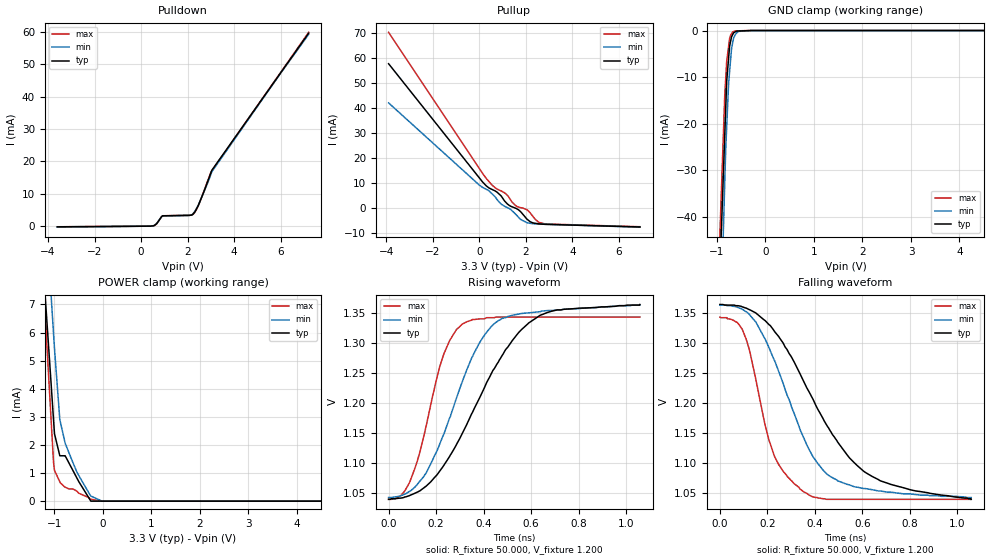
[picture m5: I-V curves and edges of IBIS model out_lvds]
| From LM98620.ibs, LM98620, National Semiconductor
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[Model] out_lvds
Model_type Output
Vref=1.20000V
Rref=50.0000ohms
Cref=0.00000F
Vmeas=1.20000V
C_comp 737.000fF 691.000fF 817.000fF
| variable typ   min   max
[Voltage Range] 3.30000V 3.00000V 3.60000V
[POWER Clamp Reference] 3.30000V 3.00000V 3.60000V
[Pullup Reference] 3.30000V 3.00000V 3.60000V
[Pulldown Reference] 0.00000V 0.00000V 0.00000V
[GND Clamp Reference] 0.00000V 0.00000V 0.00000V
[Temperature Range]   25   70   0
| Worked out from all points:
|   slope of the pulldown table from 0 to 0.495 V, typ, clamps not added: 4.65 kohm
|   slope of the pullup table from 0 to 0.495 V, typ, clamps not added: 113 ohm
|   GND clamp passes 1 mA (typ) near -0.68 V on its own axis
|   POWER clamp passes 1 mA (typ) near -0.59 V on its own axis
|   rising waveform, R_fixture 50.000, V_fixture 1.200: 20-80 % time 266ps typ, 194ps min, 115ps max; typ from 1.04 V to 1.36 V
|   falling waveform, R_fixture 50.000, V_fixture 1.200: 20-80 % time 289ps typ, 200ps min, 116ps max; typ from 1.36 V to 1.04 V
[GND Clamp]
-3.6V     -828.7mA   -1.023A    -833.8mA
-3V       -653.4mA   -808mA     -655.6mA
-840mV    -22.57mA   -32.76mA   -14mA
-820mV    -16.73mA   -25.58mA   -10.34mA
-800mV    -10.89mA   -20.83mA   -6.68mA
-760mV    -5.872mA   -11.32mA   -3.357mA
-740mV    -3.363mA   -8.853mA   -1.695mA
-700mV    -1.363mA   -3.922mA   -701.6uA
-660mV    -522.6uA   -1.717mA   -216.5uA
-560mV    -109.8uA   -188.4uA   -61.51uA
-280mV    0A         0A         0A
7.2V      0A         0A         0A
[Pulldown]
-3.6V     -228.1uA   -333.2uA   -216.3uA
400mV     -26.54uA   -21.17uA   -29.46uA
540mV     100.7uA    166uA      76.81uA
680mV     832uA      952.1uA    779.9uA
920mV     3.176mA    3.133mA    3.192mA
2.06V     3.322mA    3.282mA    3.336mA
2.22V     3.619mA    3.762mA    3.559mA
2.34V     4.764mA    4.947mA    4.614mA
2.5V      7.154mA    7.187mA    6.982mA
3V        16.5mA     16.05mA    16.71mA
3.04V     17.27mA    16.85mA    17.12mA
7.2V      59.7mA     59.34mA    59.95mA
[Pullup]
-3.9V     57.71mA    42.03mA    70.29mA
0V        12mA       9.116mA    15.74mA
260mV     9.187mA    7.62mA     12.25mA
420mV     7.937mA    6.794mA    10.47mA
760mV     6.288mA    3.336mA    7.56mA
1.12V     2.406mA    487.7uA    5.771mA
1.58V     -213.1uA   -2.707mA   748.1uA
1.78V     -1.58mA    -4.658mA   76.77uA
2.18V     -5.52mA    -6.172mA   -1.952mA
2.52V     -6.367mA   -6.468mA   -5.559mA
2.8V      -6.573mA   -6.548mA   -6.373mA
6.9V      -7.647mA   -7.716mA   -7.544mA
[POWER Clamp]
-3.9V     76.64mA    84.41mA    106.3mA
-1.3V     10.08mA    13.6mA     10.8mA
-1.16V    6.495mA    9.79mA     5.659mA
-1.02V    2.911mA    5.977mA    1.391mA
-1V       2.399mA    5.433mA    1.094mA
-890mV    1.615mA    2.904mA    689.6uA
-780mV    1.615mA    2.062mA    496.3uA
-540mV    829.4uA    1.046mA    358.3uA
-500mV    698.5uA    914.1uA    282.6uA
-250mV    0A         180.7uA    65.92uA
-20mV     0A         0A         0A
6.9V      0A         0A         0A
[Rising Waveform]
R_fixture = 50.000
V_fixture = 1.200
V_fixture_min = 1.200
V_fixture_max = 1.200
|  time   V(typ)   V(min)   V(max)
0s        1.04V      1.043V     1.04V
87ps      1.046V     1.053V     1.067V
155ps     1.061V     1.082V     1.157V
233ps     1.097V     1.149V     1.283V
309ps     1.149V     1.235V     1.332V
360ps     1.191V     1.284V     1.34V
429ps     1.247V     1.327V     1.343V
589ps     1.334V     1.351V     1.344V
710ps     1.356V     1.356V     1.344V
1.058ns   1.365V     1.364V     1.344V
[Falling Waveform]
R_fixture = 50.000
V_fixture = 1.200
V_fixture_min = 1.200
V_fixture_max = 1.200
|  time   V(typ)   V(min)   V(max)
0s        1.365V     1.364V     1.344V
94ps      1.361V     1.357V     1.324V
151ps     1.351V     1.336V     1.241V
191ps     1.338V     1.307V     1.163V
232ps     1.319V     1.27V      1.11V
355ps     1.235V     1.141V     1.052V
454ps     1.161V     1.081V     1.04V
612ps     1.085V     1.058V     1.04V
801ps     1.056V     1.049V     1.04V
1.058ns   1.04V      1.043V     1.04V
[Ramp]
dV/dt_f   1.9500E-01/2.8960E-10   1.9250E-01/1.9698E-10   1.8240E-01/1.1662E-10
dV/dt_r   1.9500E-01/2.7320E-10   1.9250E-01/1.9510E-10   1.8240E-01/1.2330E-10
R_load = 50
